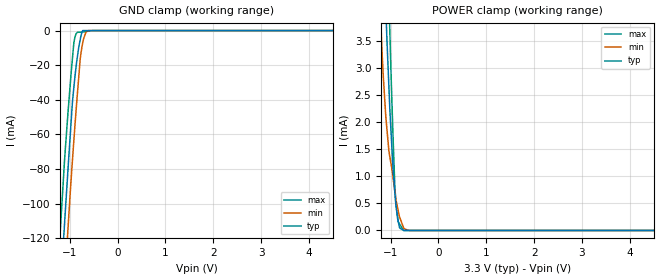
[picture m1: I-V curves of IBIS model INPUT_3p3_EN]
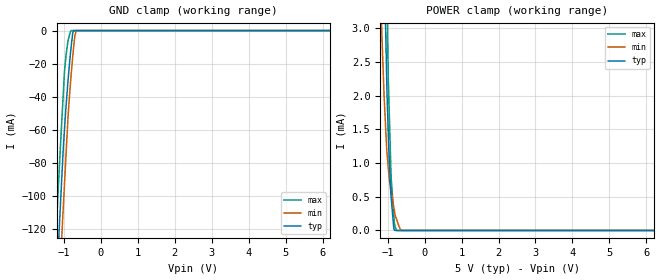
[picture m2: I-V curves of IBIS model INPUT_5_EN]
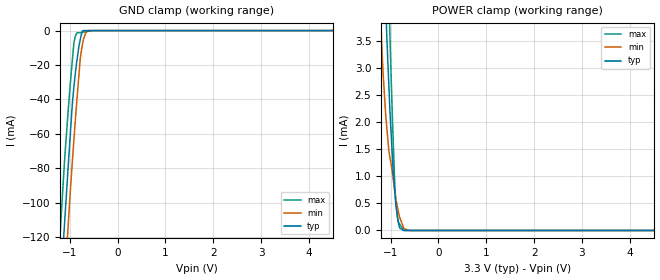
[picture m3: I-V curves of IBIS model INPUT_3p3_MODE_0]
|Texas Instruments Incorporated
|16-Bit, Serial Input Multiplying Digital to Analog Converter
| Marketing part#   Digital Voltage Range   Package-type   #pins
| DAC8811IBDGKR   2.7V to 5.5V   MSOP   8
| DAC8811IBDGKRG4   2.7V to 5.5V   MSOP   8
| DAC8811IBDGKT   2.7V to 5.5V   MSOP   8
| DAC8811IBDGKTG4   2.7V to 5.5V   MSOP   8
| DAC8811ICDGKR   2.7V to 5.5V   MSOP   8
| DAC8811ICDGKRG4   2.7V to 5.5V   MSOP   8
| DAC8811ICDGKT   2.7V to 5.5V   MSOP   8
| DAC8811ICDGKTG4   2.7V to 5.5V   MSOP   8
| DAC8811IBDRBR   2.7V to 5.5V   SON   8
| DAC8811IBDRBRG4   2.7V to 5.5V   SON   8
| DAC8811IBDRBT   2.7V to 5.5V   SON   8
| DAC8811IBDRBTG4   2.7V to 5.5V   SON   8
| DAC8811ICDRBR   2.7V to 5.5V   SON   8
| DAC8811ICDRBRG4   2.7V to 5.5V   SON   8
| DAC8811ICDRBT   2.7V to 5.5V   SON   8
| DAC8811ICDRBTG4   2.7V to 5.5V   SON   8
[IBIS Ver]   3.2
[File name]   dac8811.ibs
|SIMDE Ver   V2.0 - 201002 - RHL4 - Build 372
[Date]   08/30/2010
[File Rev]   1.2
[Source]
| Texas Instruments Incorporated.
| Analog eLab Design Center, HPA
| 12500 TI Blvd
| Dallas, TX -75243
| e-Mail: elab_scm_ibis@list.ti.com
| Model generated from simulations in TISPICE
[Notes]   Revision_History:
|   Rev 1.0: 07/26/2010
|   - Initial version of the model
|   - Model names with a trailing _3p3 contains the model for
|   3V [3 - 3.3 - 3.6]. Model names with trailing _5 contains
|   the model for 5V [4.5 - 5.0 - 5.5] operation.
|   - Model generated from simulations in TISPICE
|   - Model matched to SPICE simulation
|   - While calculating R_pkg, L_pkg and C_pkg ignored values
|   corresponding to power and ground pins
|   - Added package details beside [Package]
|   - C_comp although listed in numerical order of value are
|   obtained from varying PVT conditions. For PVT conditions
|   for each specific value refer the buffer description under
|   respective [Model]. IBIS model user is responsible for using
|   appropriate C_comp to simulate for Signal Integrity.
|   Rev 1.1: 08/03/2010
|   - Updated ibis file format for multiple packages
|   Rev 1.2: 08/30/2010
|   - Updated the ibis file specified by TI for multiple modes
|   and added TERM model
[Disclaimer]
| This model is designed as an aid for customers of Texas Instruments.
| TI and its licensors and suppliers make no warranties, either expressed
| or implied, with respect to this  model, including the warranties of
| merchantability or fitness for a particular purpose. The model is
| provided solely on an "as is" basis. The entire risk as to its quality
| and performance is with the customer.
[Copyright]
| (C) Copyright 2010 Texas Instruments Incorporated. All rights reserved.
|   DAC8811IBDGK
[Component]   DAC8811IBDGK
[Manufacturer]  TI
[Package]  | 8 SON   - DGK package
| variable   typ   min   max
R_pkg   0.03162   0.01831   0.04135
L_pkg   1.30962nH   1.09430nH   1.47824nH
C_pkg   0.30988pF   0.28453pF   0.35235pF
|-------------------------PIN------------------------------------------------
[Pin]  signal_name model_name   R_pin   L_pin   C_pin
1   CLK   INPUT_EN   0.03716   1.36302nH   0.28453pF
2   SDI   INPUT_MODE   0.03439   1.27538nH   0.32677pF
3   RFB   TERM   0.01831   1.09430nH   0.35235pF
4   VREF   TERM   0.02161   1.29118nH   0.31446pF
5   IOUT   TERM   0.04135   1.47824nH   0.29456pF
6   GND   GND   0.01346   1.09004nH   0.36449pF
7   VDD   POWER   0.01772   1.07679nH   0.34588pF
8   _CS   INPUT_EN   0.03687   1.35560nH   0.28660pF
|   DAC8811ICDGK
[Component]   DAC8811ICDGK
[Manufacturer]  TI
[Package]  | 8 SON   - DGK package
| variable   typ   min   max
R_pkg   0.03162   0.01831   0.04135
L_pkg   1.30962nH   1.09430nH   1.47824nH
C_pkg   0.30988pF   0.28453pF   0.35235pF
|-------------------------PIN------------------------------------------------
[Pin]  signal_name model_name   R_pin   L_pin   C_pin
1   CLK   INPUT_EN   0.03716   1.36302nH   0.28453pF
2   SDI   INPUT_MODE   0.03439   1.27538nH   0.32677pF
3   RFB   TERM   0.01831   1.09430nH   0.35235pF
4   VREF   TERM   0.02161   1.29118nH   0.31446pF
5   IOUT   TERM   0.04135   1.47824nH   0.29456pF
6   GND   GND   0.01346   1.09004nH   0.36449pF
7   VDD   POWER   0.01772   1.07679nH   0.34588pF
8   _CS   INPUT_EN   0.03687   1.35560nH   0.28660pF
|   DAC8811IBDRB
[Component]   DAC8811IBDRB
[Manufacturer]  TI
[Package]  | 8 SON   - DRB package
| variable   typ   min   max
R_pkg   0.03301   0.01850   0.04292
L_pkg   0.83135nH   0.60811nH   0.99618nH
C_pkg   0.11016pF   0.09713pF   0.12927pF
|-------------------------PIN------------------------------------------------
[Pin]  signal_name model_name   R_pin   L_pin   C_pin
1   CLK   INPUT_EN   0.03929   0.89418nH   0.09713pF
2   SDI   INPUT_MODE   0.03703   0.83551nH   0.10036pF
3   RFB   TERM   0.01850   0.60811nH   0.12855pF
4   VREF   TERM   0.02126   0.76638nH   0.12927pF
5   IOUT   TERM   0.04292   0.99618nH   0.10656pF
6   GND   GND   0.01277   0.59237nH   0.14229pF
7   VDD   POWER   0.01803   0.59604nH   0.12276pF
8   _CS   INPUT_EN   0.03904   0.88774nH   0.09911pF
|   DAC8811ICDRB
[Component]   DAC8811ICDRB
[Manufacturer]  TI
[Package]  | 8 SON   - DRB package
| variable   typ   min   max
R_pkg   0.03301   0.01850   0.04292
L_pkg   0.83135nH   0.60811nH   0.99618nH
C_pkg   0.11016pF   0.09713pF   0.12927pF
|-------------------------PIN------------------------------------------------
[Pin]  signal_name model_name   R_pin   L_pin   C_pin
1   CLK   INPUT_EN   0.03929   0.89418nH   0.09713pF
2   SDI   INPUT_MODE   0.03703   0.83551nH   0.10036pF
3   RFB   TERM   0.01850   0.60811nH   0.12855pF
4   VREF   TERM   0.02126   0.76638nH   0.12927pF
5   IOUT   TERM   0.04292   0.99618nH   0.10656pF
6   GND   GND   0.01277   0.59237nH   0.14229pF
7   VDD   POWER   0.01803   0.59604nH   0.12276pF
8   _CS   INPUT_EN   0.03904   0.88774nH   0.09911pF
|   Model Selectors
[Model Selector]  INPUT_EN
INPUT_3p3_EN   3V digital input
INPUT_5_EN   5V digital input
|NOTES   Model INPUT_EN split into two Models INPUT_3p3_EN and INPUT_5_EN
|   to accomodate vast voltage range of 2.7V - 5.5V
|   INPUT_3p3_EN operates in voltage range of 3.0 - 3.3 - 3.6
|   INPUT_5_EN operates in voltage range of 4.5 - 5.0 - 5.5
|   The min pin frequency for Model INPUT_EN is 50MHz
|   This is referenced with datasheet
[Model Selector]  INPUT_MODE
INPUT_3p3_MODE_0  3V digital input
INPUT_5_MODE_0   5V digital input
|NOTES   Model INPUT_MODE split into two Models INPUT_3p3_MODE_0 and
|   INPUT_5_MODE_0 to accomodate vast voltage range of 2.7V - 5.5V
|   INPUT_3p3_MODE_0 operates in voltage range of 3.0 - 3.3 - 3.6
|   INPUT_5_MODE_0 operates in voltage range of 4.5 - 5.0 - 5.5
|   The min pin frequency for Model INPUT_MODE is 25MHz
|   This is referenced with datasheet
[Model selector] TERM
TERM_3p3  3.3V nominal termination
TERM_5   5.0V nominal termination
|   Termination - TERM_3p3
[Model] TERM_3p3
Model_type Terminator
C_comp   1.0e-20F  1.0e-20F  1.0e-20F
| variable   typ   min   max
[Voltage Range]   3.3   3   3.6
[Power Clamp Reference]   3.3   3   3.6
[GND Clamp Reference]   0   0   0
|Ambient Temperature   25   85   -40
|Junction Temperature
[Temperature Range]   26   86   -40
|   Termination - TERM_5
[Model] TERM_5
Model_type Terminator
C_comp   1.0e-20F  1.0e-20F  1.0e-20F
| variable   typ   min   max
[Voltage Range]   5   4.5   5.5
[Power Clamp Reference]   5   4.5   5.5
[GND Clamp Reference]   0   0   0
|Ambient Temperature   25   85   -40
|Junction Temperature
[Temperature Range]   26   86   -40
| Models and submodels in the file (6): INPUT_3p3_EN (Input), INPUT_5_EN (Input), INPUT_3p3_MODE_0 (Input), INPUT_5_MODE_0 (Input), TERM_3p3 (Terminator), TERM_5 (Terminator)
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|   Input INPUT_EN 3V Model
[Model] INPUT_3p3_EN
Model_type Input
| Signals   CLK(1), _CS(8)
Vinl = 0.6
Vinh = 2.1
|   typ   min   max
|   (nom PVT)   (Fast PVT)   (slow PVT)
C_comp   9.251e-13   9.181e-13   9.473e-13
| Where   nom PVT is  Nominal Process, 3.3V, 26C
|   Fast PVT is Strong Process, 3.6V, -40C
|   Slow PVT is Weak Process, 3.0V, 86C
[Voltage Range]   3.3   3   3.6
|Ambient Temperature   25   85   -40
|Junction Temperature
[Temperature Range]   26   86   -40
[Power Clamp Reference]   3.3   3   3.6
[GND Clamp Reference]   0   0   0
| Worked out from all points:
|   GND clamp passes 1 mA (typ) near -0.74 V on its own axis
|   POWER clamp passes 1 mA (typ) near -0.94 V on its own axis
[GND Clamp]
|   Voltage   I(typ)   I(min)   I(max)
-3.3V     -1.185A    -1.216A    -1.155A
-1.211V   -158.6mA   -194mA     -122.2mA
-1.18V    -144mA     -179.4mA   -107.6mA
-1.111V   -113mA     -148.2mA   -76.34mA
-1.036V   -80.07mA   -114.3mA   -47.16mA
-947.1mV  -42.84mA   -76.61mA   -17.4mA
-913.2mV  -32.71mA   -63.4mA    -6.977mA
-841.2mV  -15.42mA   -37.14mA   -990.8uA
-780mV    -5.101mA   -16.22mA   -962.1uA
-744mV    -1.13mA    -9.375mA   -801.3uA
-615mV    0A         0A         -377.9uA
6.6V      0A         0A         0A
[POWER Clamp]
|   Voltage   I(typ)   I(min)   I(max)
-3.3V     92.74mA    75.13mA    116.7mA
-1.244V   8.697mA    4.794mA    12.99mA
-1.188V   6.727mA    3.499mA    10.45mA
-1.095V   3.984mA    2.045mA    6.361mA
-1.076V   3.501mA    1.859mA    5.68mA
-1.016V   2.249mA    1.361mA    3.685mA
-949.2mV  1.138mA    971.2uA    1.743mA
-913.2mV  727.7uA    731.5uA    849.9uA
-891.6mV  495.6uA    590.6uA    548.7uA
-841.2mV  165.6uA    364.4uA    165uA
-729.6mV  1.861uA    52.37uA    0A
6.6V      0A         0A         0A
|   Input INPUT_EN 5V Model
[Model] INPUT_5_EN
Model_type Input
| Signals   CLK(1), _CS(8)
Vinl = 0.8
Vinh = 2.4
|   typ   min   max
|   (nom PVT)   (Fast PVT)   (slow PVT)
C_comp   8.580e-13   8.507e-13   8.809e-13
| Where   nom PVT is  Nominal Process, 5.0V, 26C
|   Fast PVT is Strong Process, 5.5V, -40C
|   Slow PVT is Weak Process, 4.5V, 86C
[Voltage Range]   5   4.5   5.5
|Ambient Temperature   25   85   -40
|Junction Temperature
[Temperature Range]   26   86   -40
[Power Clamp Reference]   5   4.5   5.5
[GND Clamp Reference]   0   0   0
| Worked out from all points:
|   GND clamp passes 1 mA (typ) near -0.75 V on its own axis
|   POWER clamp passes 1 mA (typ) near -0.95 V on its own axis
[GND Clamp]
|   Voltage   I(typ)   I(min)   I(max)
-5V       -2.035A    -2.063A    -2.009A
-1.21V    -158mA     -193.7mA   -121.4mA
-1.15V    -130.6mA   -165.8mA   -94.27mA
-1.115V   -114.7mA   -150.2mA   -79.16mA
-1.073V   -96.09mA   -131.6mA   -61.09mA
-1.022V   -73.45mA   -109mA     -40.16mA
-941mV    -45.61mA   -74.28mA   -14.66mA
-887mV    -29.63mA   -51.66mA   -6.049mA
-801.5mV  -9.25mA    -25.88mA   0A
-750mV    -587.4uA   -13.03mA   0A
-662mV    0A         0A         0A
10V       0A         0A         0A
[POWER Clamp]
|   Voltage   I(typ)   I(min)   I(max)
-5V       164.4mA    136.5mA    204.1mA
-1.161V   5.956mA    3.003mA    9.27mA
-1.099V   4.17mA     2.02mA     6.677mA
-1.056V   3.055mA    1.547mA    4.949mA
-1.015V   1.991mA    1.128mA    3.399mA
-970mV    1.23mA     848.6uA    1.994mA
-925mV    650.3uA    653.5uA    1.128mA
-902.5mV  466.8uA    578.2uA    762.5uA
-835mV    37.17uA    352.2uA    233.3uA
-797mV    0A         225uA      47.93uA
-639.5mV  0A         0A         0A
10V       0A         0A         0A
|   Input INPUT_MODE 3V Model
[Model] INPUT_3p3_MODE_0
Model_type Input
| Signals   SDI(2)
Vinl = 0.6
Vinh = 2.1
|   typ   min   max
|   (nom PVT)   (Fast PVT)   (slow PVT)
C_comp   1.006e-12   9.999e-13   1.028e-12
| Where   nom PVT is  Nominal Process, 3.3V, 26C
|   Fast PVT is Strong Process, 3.6V, -40C
|   Slow PVT is Weak Process, 3.0V, 86C
[Voltage Range]   3.3   3   3.6
|Ambient Temperature   25   85   -40
|Junction Temperature
[Temperature Range]   26   86   -40
[Power Clamp Reference]   3.3   3   3.6
[GND Clamp Reference]   0   0   0
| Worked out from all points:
|   GND clamp passes 1 mA (typ) near -0.74 V on its own axis
|   POWER clamp passes 1 mA (typ) near -0.94 V on its own axis
[GND Clamp]
|   Voltage   I(typ)   I(min)   I(max)
-3.3V     -1.189A    -1.22A     -1.16A
-1.214V   -160.9mA   -196.4mA   -124.5mA
-1.187V   -148.1mA   -183.5mA   -111.7mA
-1.111V   -113.6mA   -149mA     -76.97mA
-1.044V   -84.19mA   -118.6mA   -50.93mA
-947.1mV  -43.2mA    -77.01mA   -17.8mA
-913.2mV  -33.04mA   -63.76mA   -7.335mA
-841.2mV  -15.61mA   -37.37mA   -1.254mA
-780mV    -5.263mA   -16.41mA   -1.204mA
-750mV    -1.766mA   -10.53mA   -1.026mA
-615mV    0A         0A         -426.7uA
6.6V      0A         0A         0A
[POWER Clamp]
|   Voltage   I(typ)   I(min)   I(max)
-3.3V     92.74mA    75.13mA    116.7mA
-1.244V   8.697mA    4.794mA    12.99mA
-1.188V   6.727mA    3.499mA    10.45mA
-1.098V   4.06mA     2.081mA    6.468mA
-1.076V   3.501mA    1.863mA    5.68mA
-1.016V   2.249mA    1.356mA    3.685mA
-949.2mV  1.138mA    971.2uA    1.742mA
-913.2mV  727.7uA    731.5uA    849.9uA
-891.6mV  495.6uA    590.6uA    548.7uA
-841.2mV  165.6uA    364.4uA    165uA
-729.6mV  1.85uA     52.36uA    0A
6.6V      0A         0A         0A
